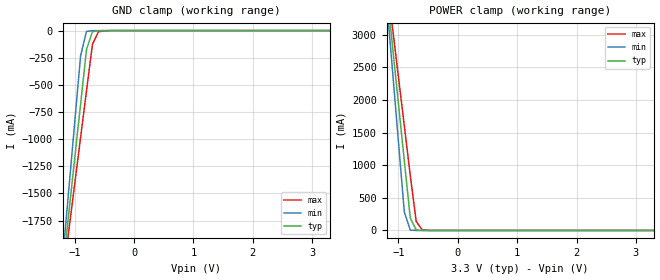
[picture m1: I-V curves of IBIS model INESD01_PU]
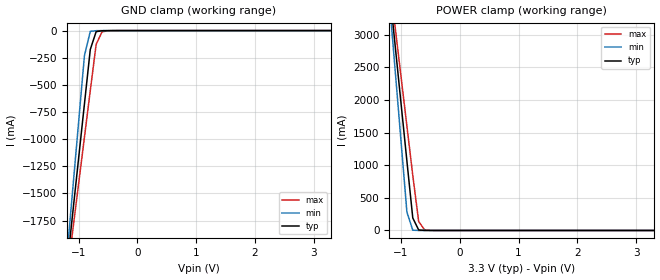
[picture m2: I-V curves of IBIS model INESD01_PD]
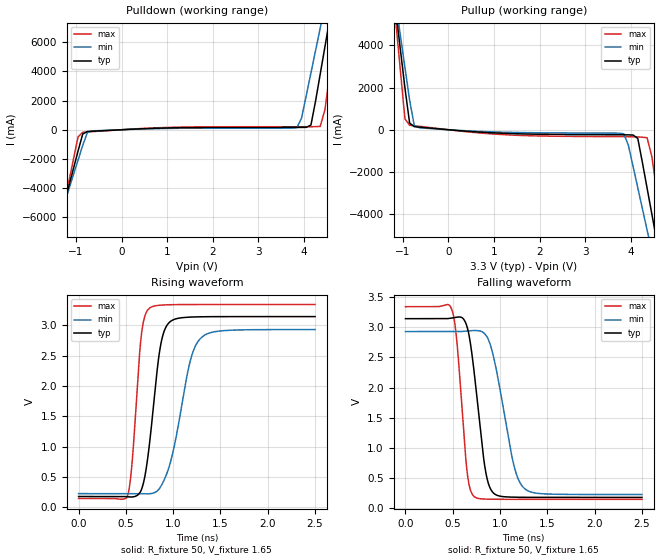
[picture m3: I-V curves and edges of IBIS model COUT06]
|   This file is an IBIS representation of the   |
|   Integrated Devices Technology, Inc.   |
|   ICS8432-111   |
|   700MHZ/350MHZ, DIFFERENTIAL-TO-3.3V  LVPECL FREQUENCY SYNTHESIZER   |
[IBIS Ver]   4.1
[File name]   8432_111_3v3.ibs
[File Rev]   1.0
[Date]   31 Dec 2008 | Last modified
|   15 Apr 2003 | Generated
[Source]   Originated at Integrated Devices Technology, Inc.
[Disclaimer]
IDT hereby grants the user of this IBIS model a non-exclusive,
nontransferable license to use this IBIS model under the following terms.
Before using this IBIS model, the user should read this license.
If the user does not accept these terms,  the IBIS model should be
returned to IDT within 30 days.
   The user is granted this license only to use the IBIS model and
is not granted rights to sell, load, rent, lease or license the IBIS
model in whole or in part, or in modified form to anyone other than
user. User may modify the IBIS model to suit its specific
applications but rights to derivative works and such modifications
shall belong to IDT.
   This IBIS model is provided on an "AS IS" basis and IDT makes
absolutely no warranty with respect to the information contained
herein. IDT DISCLAIMS AND CUSTOMER WAIVES ALL WARRANTIES, EXPRESS
OR IMPLIED, INCLUDING WARRANTIES OF MERCHANTABILITY OR FITNESS FOR
A PARTICULAR PURPOSE. The entire risk as to quality and performance
is with the Customer. ACCORDINGLY, IN NO EVENT SHALL THE COMPANY BE
LIABLE FOR ANY DAMAGES, WHETHER IN CONTRACT OR TORT,INCLUDING ANY
LOST PROFITS OR OTHER INCIDENTAL, CONSEQUENTIAL, EXEMPLARY, OR
PUNITIVE DAMAGES ARISING OUT OF THE USE OR APPLICATION OF THE IBIS
model provided in this package. Further, IDT reserves the right to
make changes without notice to any product herein to improve
reliability, function, or design. IDT does not convey any license
under patent rights or any other intellectual property rights,
including those of third parties.
   IDT is not obligated to provide maintenance or support
for the licensed IBIS model.
[Copyright]   Copyright 2003 by Integrated Devices Technology, Inc.
[Component]   ICS8432-111
[Manufacturer] Integrated Devices Technology, Inc.
[Package]
|LQFP32
|lead+wire  typ   min   max
R_pkg   220.4m   212.5m   238m
L_pkg   1.841n   1.708n   1.974n
C_pkg   0.316p   0.2907p   0.33p
[Pin]   signal_name   model_name   R_pin   L_pin   C_pin
1   M5   INESD01_PU   238m   1.974n   0.330p
2   M6   INESD01_PD   225m   1.841n   0.311p
3   M7   INESD01_PD   218m   1.7745n   0.301p
4   M8   INESD01_PD   213m   1.708n   0.291p
5   NO   INESD01_PD   213m   1.708n   0.291p
6   N1   INESD01_PD   218m   1.7745n   0.301p
7   NC   NC   225m   1.841n   0.311p
8   VEE   GND   238m   1.974n   0.330p
9   TEST   COUT06   238m   1.974n   0.330p
10   VCC   POWER   225m   1.841n   0.311p
11   FOUT/2   ONF01_PECL01_ABI   218m   1.7745n   0.301p
12   nFOUT/2   ONF01_PECL01_ABI   213m   1.708n   0.291p
13   VCCO   POWER   213m   1.708n   0.291p
14   FOUT   ONF01_PECL01_ABI   218m   1.7745n   0.301p
15   nFOUT   ONF01_PECL01_ABI   225m   1.841n   0.311p
16   VEE   GND   238m   1.974n   0.330p
17   MR   INESD01_PD   238m   1.974n   0.330p
18   S_CLOCK   INESD01_PD   225m   1.841n   0.311p
19   S_DATA   INESD01_PD   218m   1.7745n   0.301p
20   S_LOAD   INESD01_PD   213m   1.708n   0.291p
21   VCCA   POWER   213m   1.708n   0.291p
22   CLK_SEL   INESD01_PU   218m   1.7745n   0.301p
23   TEST_CLK   INESD01_PD   225m   1.841n   0.311p
24   CLK   INESD01_PD   238m   1.974n   0.330p
25   nCLK   INESD01_PU   238m   1.974n   0.330p
26   nP_LOAD   INESD01_PD   225m   1.841n   0.311p
27   VCO_SEL   INESD01_PU   218m   1.7745n   0.301p
28   M0   INESD01_PD   213m   1.708n   0.291p
29   M1   INESD01_PD   213m   1.708n   0.291p
30   M2   INESD01_PD   218m   1.7745n   0.301p
31   M3   INESD01_PD   225m   1.841n   0.311p
32   M4   INESD01_PD   238m   1.974n   0.330p
[Diff Pin]  inv_pin  vdiff tdelay_typ tdelay_min  tdelay_max
11   12   NA   0  0  0
14   15   NA   0  0  0
24   25   0.15 0  0  0
| Models and submodels in the file (4): INESD01_PU (Input), INESD01_PD (Input), COUT06 (Output), ONF01_PECL01_ABI (Output_ECL)
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[Model]   INESD01_PU
Model_type   Input
Polarity   Non-Inverting
Vinl = 0.8V
Vinh = 2.0V
|   typ   min   max
C_comp   2pF   1.5pF   2.5pF
|   typ   min   max
[Voltage range]  3.3V   3.15V   3.45V
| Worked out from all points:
|   GND clamp passes 1 mA (typ) near -0.55 V on its own axis
|   POWER clamp passes 1 mA (typ) near -0.61 V on its own axis
[GND_clamp]
|Voltage   I(typ)   I(min)   I(max)
-3.3V     -12.83A    -15.14A    -11.37A
-1.2V     -2.195A    -2.092A    -2.281A
-1.1V     -1.689A    -1.472A    -1.849A
-900mV    -678.5mA   -232.7mA   -984.8mA
-800mV    -174mA     -7.237mA   -553.3mA
-700mV    -9.767mA   -1.114mA   -126.1mA
-600mV    -1.7mA     -240.1uA   -11.15mA
-300mV    -81.66uA   -67.79uA   -163.4uA
3.3V      1.866nA    1.113pA    239.1nA
[POWER_clamp]
|Voltage   I(typ)   I(min)   I(max)
-3.3V     22.38A     26.45A     19.82A
-1.2V     3.723A     3.545A     3.874A
-1.1V     2.836A     2.457A     3.116A
-1V       1.949A     1.369A     2.358A
-900mV    1.063A     281mA      1.601A
-800mV    191.5mA    5.012mA    843.9mA
-700mV    8.032mA    142.2uA    138.3mA
-600mV    607uA      17.63uA    10.62mA
-400mV    16.32uA    7.545uA    335.9uA
3.3V      -71.13uA   -62.11uA   -78.26uA
[Model]   INESD01_PD
Model_type   Input
Polarity   Non-Inverting
Vinl = 0.80V
Vinh = 2.0V
|   typ   min   max
C_comp   2pF   1.5pF   2.5pF
|   typ   min   max
[Voltage range]  3.3V   3.15V   3.45V
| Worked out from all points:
|   GND clamp passes 1 mA (typ) near -0.55 V on its own axis
|   POWER clamp passes 1 mA (typ) near -0.60 V on its own axis
[GND_clamp]
|Voltage I(typ)   I(min)   I(max)
-3.3V     -12.83A    -15.14A    -11.37A
-1.2V     -2.195A    -2.092A    -2.281A
-1.1V     -1.689A    -1.472A    -1.849A
-900mV    -678.5mA   -232.6mA   -984.8mA
-800mV    -173.9mA   -7.175mA   -553.2mA
-700mV    -9.696mA   -1.052mA   -126mA
-600mV    -1.629mA   -178uA     -11.07mA
-300mV    -10.53uA   -5.678uA   -86.08uA
3.3V      71.13uA    62.11uA    77.58uA
[POWER_clamp]
|Voltage   I(typ)   I(min)   I(max)
-3.3V     22.38A     26.45A     19.82A
-1.2V     3.723A     3.545A     3.874A
-1.1V     2.836A     2.457A     3.116A
-1V       1.949A     1.369A     2.358A
-900mV    1.063A     281.1mA    1.601A
-800mV    191.6mA    5.074mA    844mA
-700mV    8.104mA    204.3uA    138.4mA
-600mV    678.1uA    79.74uA    10.7mA
-400mV    87.44uA    69.65uA    413.2uA
3.3V      -3.041nA   -425fA     -919.9nA
[Model]   COUT06
Model_type   Output
Polarity   Non-Inverting
|   typ   min   max
C_comp   2pF   1.5pF   2.5pF
Vmeas = 1.65V
Rref = 50
Vref = 1.65V
|   typ   min   max
[Voltage range]   3.3V   3.135V   3.465V
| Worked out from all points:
|   slope of the pulldown table from 0 to 0.495 V, typ, clamps not added: 6.88 ohm
|   slope of the pullup table from 0 to 0.495 V, typ, clamps not added: 5.83 ohm
|   rising waveform, R_fixture 50, V_fixture 1.65: 20-80 % time 127ps typ, 201ps min, 86.3ps max; typ from 0.181 V to 3.14 V
|   falling waveform, R_fixture 50, V_fixture 1.65: 20-80 % time 128ps typ, 189ps min, 92.7ps max; typ from 3.14 V to 0.181 V
[pulldown]
|Voltage   I (typ)   I (min)   I (max)
-3.3V     -29.26A    -25.24A    -35.98A
-1.463V   -7.508A    -7.113A    -8.217A
-1.361V   -6.298A    -6.106A    -6.67A
-952.6mV  -1.454A    -2.076A    -481.7mA
-850.5mV  -293.8mA   -1.069A    -175.5mA
-646.4mV  -102mA     -81.18mA   -129.6mA
3.844V    159mA      144.7mA    203.8mA
4.151V    319.9mA    3.884A     206.6mA
4.355V    3.815A     6.961A     228.9mA
4.559V    7.514A     10.04A     3.725A
4.763V    11.22A     13.12A     8.46A
6.6V      44.81A     41.05A     51.4A
[pullup]
|Voltage   I (typ)   I (min)   I (max)
-3.3V     44.73A     38.54A     55.09A
-1.157V   5.7A       6.046A     5.224A
-1.055V   3.84A      4.498A     2.846A
-952.6mV  1.979A     2.95A      516.9mA
-850.5mV  318.6mA    1.402A     214.1mA
-748.5mV  147.6mA    205.9mA    188.2mA
3.844V    -239.7mA   -193.2mA   -328.3mA
4.151V    -416.1mA   -2.755A    -342.5mA
4.355V    -2.772A    -4.758A    -379.9mA
4.559V    -5.183A    -6.764A    -2.792A
4.763V    -7.594A    -8.771A    -5.873A
6.6V      -29.3A     -26.85A    -33.6A
[Ramp]
|   typ   min   max
dV/dt_r   2.374/0.197n   2.162/0.318n   2.564/0.133n
dV/dt_f   2.390/0.193n   2.173/0.283n   2.581/0.140n
[Rising Waveform]
R_fixture = 50
V_fixture = 1.65
V_fixture_max = 1.7325
V_fixture_min = 1.56
C_fixture = 0.0p
| Time   typ   min   max
0s        180.7mV    228.1mV    148.5mV
517.1ps   175.7mV    228.2mV    190.5mV
564.8ps   172.8mV    228.4mV    725.4mV
662.6ps   287.2mV    227.2mV    2.825V
748ps     1.026V     225.5mV    3.276V
863.4ps   2.637V     331.6mV    3.328V
971.4ps   3.061V     746.1mV    3.336V
1.175ns   3.132V     2.376V     3.339V
1.298ns   3.137V     2.795V     3.339V
2.5ns     3.141V     2.927V     3.339V
[Falling Waveform]
R_fixture = 50
V_fixture = 1.65
V_fixture_max = 1.7325
V_fixture_min = 1.56
C_fixture = 0.0p
| Time   typ   min   max
0s        3.141V     2.927V     3.339V
489.5ps   3.152V     2.927V     3.292V
542.2ps   3.165V     2.927V     2.783V
652.6ps   2.999V     2.936V     592.4mV
727.9ps   2.231V     2.945V     192.6mV
828.3ps   806.2mV    2.905V     153.4mV
888.5ps   358.5mV    2.748V     150.6mV
1.142ns   184.2mV    738.8mV    148.6mV
1.252ns   181.9mV    336.5mV    148.5mV
2.5ns     180.7mV    228.1mV    148.5mV
